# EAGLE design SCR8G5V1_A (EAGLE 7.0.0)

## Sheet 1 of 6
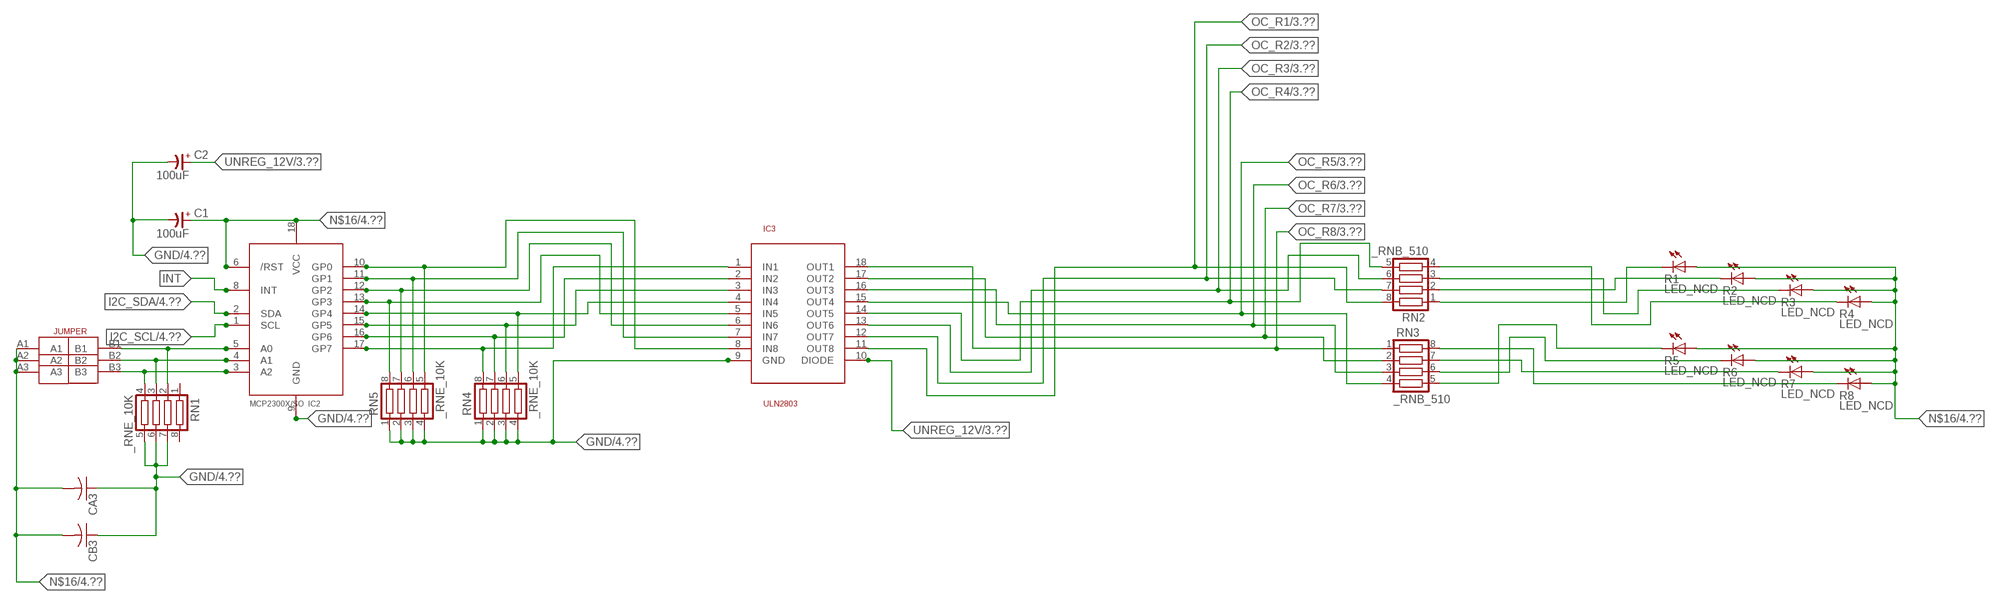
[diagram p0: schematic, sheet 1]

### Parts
C1  100uF  CP-E-025X060  [E-025X060]
C2  100uF  CP-E-025X060  [E-025X060]
CA3  CC1206KRX7R9BB104C1206K  [CC1206KRX7R9BB104]
CB3  TMK316F106ZL-TC1206K  [TMK316F106ZL-T]
IC2  MCP2300X/SO  [SO18W]
IC3  ULN2803  [SO18L]
R1  LED_NCD  [CHIPLED_0603]
R2  LED_NCD  [CHIPLED_0603]
R3  LED_NCD  [CHIPLED_0603]
R4  LED_NCD  [CHIPLED_0603]
R5  LED_NCD  [CHIPLED_0603]
R6  LED_NCD  [CHIPLED_0603]
R7  LED_NCD  [CHIPLED_0603]
R8  LED_NCD  [CHIPLED_0603]
RN1  _RNE_10K  [RNE]
RN2  _RNB_510  [RNB]
RN3  _RNB_510  [RNB]
RN4  _RNE_10K  [RNE]
RN5  _RNE_10K  [RNE]
U$18  JUMPER_3X2  [JUMPER_3X2]

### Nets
GND: C1.- C2.- CA3.1 CB3.1 IC2.9(GND) IC3.9(GND) RN1.5 RN1.6 RN1.7 RN4.1 RN4.2 RN4.3 RN4.4 RN5.1 RN5.2 RN5.3 RN5.4 ; also sheet 4,6
GP4: IC2.14(GP4) IC3.4(IN4) RN4.5
GP6: IC2.16(GP6) IC3.2(IN2) RN4.7
I2C_SCL: IC2.1(SCL) ; also sheet 4
I2C_SDA: IC2.2(SDA) ; also sheet 4
INT: IC2.8(INT)
N$6: IC2.5(A0) RN1.2 U$18.B1
N$7: IC2.4(A1) RN1.3 U$18.B2
N$8: IC2.3(A2) RN1.4 U$18.B3
N$16: C1.+ CA3.2 CB3.2 IC2.6(/RST) IC2.18(VCC) R1.A R2.A R3.A R4.A R5.A R6.A R7.A R8.A U$18.A1 U$18.A2 U$18.A3 ; also sheet 4,6
N$20: R1.C RN2.1
N$21: IC2.12(GP2) IC3.6(IN6) RN5.7
N$22: IC2.11(GP1) IC3.7(IN7) RN5.6
N$23: IC2.10(GP0) IC3.8(IN8) RN5.5
N$29: R2.C RN2.2
N$30: R3.C RN2.3
N$31: R4.C RN2.4
N$32: R8.C RN3.8
N$81: R7.C RN3.7
N$82: R6.C RN3.6
N$83: R5.C RN3.5
N$89: IC2.13(GP3) IC3.5(IN5) RN5.8
N$93: IC2.15(GP5) IC3.3(IN3) RN4.6
N$94: IC2.17(GP7) IC3.1(IN1) RN4.8
OC_R1: IC3.11(OUT8) RN2.8 ; also sheet 3
OC_R2: IC3.12(OUT7) RN2.7 ; also sheet 3
OC_R3: IC3.13(OUT6) RN2.6 ; also sheet 3
OC_R4: IC3.14(OUT5) RN2.5 ; also sheet 3
OC_R5: IC3.15(OUT4) RN3.4 ; also sheet 3
OC_R6: IC3.16(OUT3) RN3.3 ; also sheet 3
OC_R7: IC3.17(OUT2) RN3.2 ; also sheet 3
OC_R8: IC3.18(OUT1) RN3.1 ; also sheet 3
UNREG_12V: C2.+ IC3.10(DIODE) ; also sheet 3,4
Unconnected: RN1.1 RN1.8

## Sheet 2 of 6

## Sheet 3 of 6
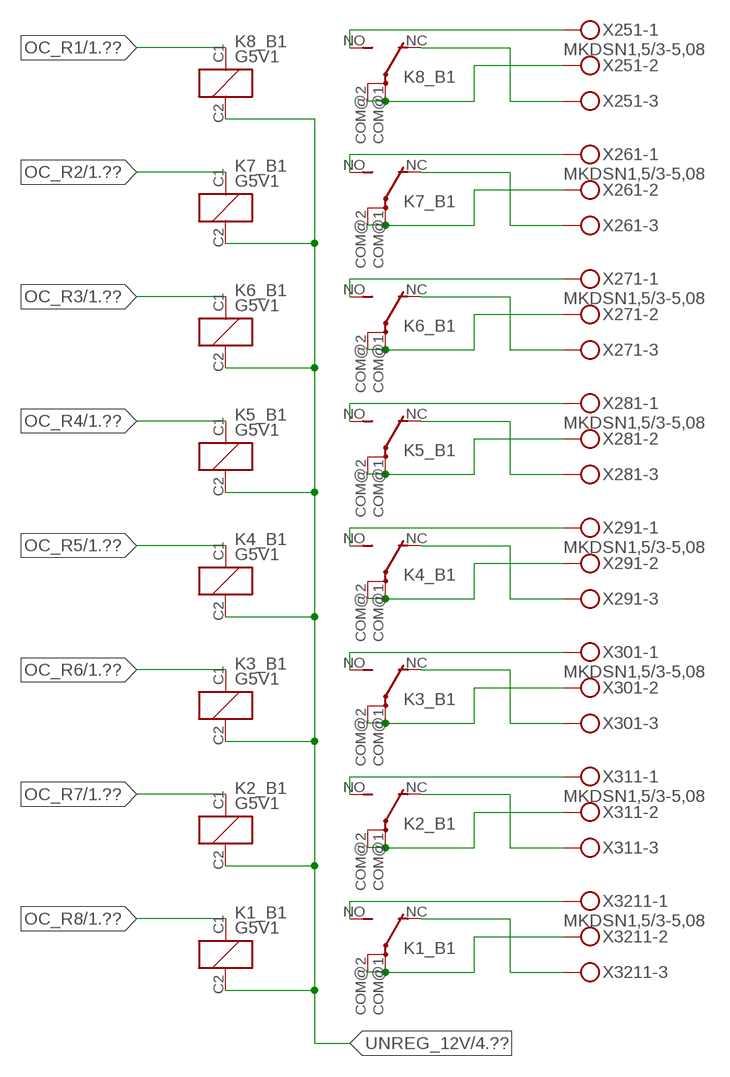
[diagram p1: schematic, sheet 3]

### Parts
K1_B1  G5V1  [G5V1]
K2_B1  G5V1  [G5V1]
K3_B1  G5V1  [G5V1]
K4_B1  G5V1  [G5V1]
K5_B1  G5V1  [G5V1]
K6_B1  G5V1  [G5V1]
K7_B1  G5V1  [G5V1]
K8_B1  G5V1  [G5V1]
X251  MKDSN1,5/3-5,08  [MKDSN1,5/3-5,08]
X261  MKDSN1,5/3-5,08  [MKDSN1,5/3-5,08]
X271  MKDSN1,5/3-5,08  [MKDSN1,5/3-5,08]
X281  MKDSN1,5/3-5,08  [MKDSN1,5/3-5,08]
X291  MKDSN1,5/3-5,08  [MKDSN1,5/3-5,08]
X301  MKDSN1,5/3-5,08  [MKDSN1,5/3-5,08]
X311  MKDSN1,5/3-5,08  [MKDSN1,5/3-5,08]
X3211  MKDSN1,5/3-5,08  [MKDSN1,5/3-5,08]

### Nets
N$203: K8_B1.COM@1(2:P) K8_B1.COM@2(2:P) X251.2
N$204: K8_B1.NC(2:O) X251.3
N$205: K8_B1.NO(2:S) X251.1
N$206: K7_B1.NO(2:S) X261.1
N$207: K6_B1.NO(2:S) X271.1
N$208: K7_B1.NC(2:O) X261.3
N$209: K7_B1.COM@1(2:P) K7_B1.COM@2(2:P) X261.2
N$210: K6_B1.NC(2:O) X271.3
N$211: K6_B1.COM@1(2:P) K6_B1.COM@2(2:P) X271.2
N$212: K5_B1.NC(2:O) X281.3
N$213: K5_B1.COM@1(2:P) K5_B1.COM@2(2:P) X281.2
N$214: K5_B1.NO(2:S) X281.1
N$215: K4_B1.NO(2:S) X291.1
N$216: K4_B1.NC(2:O) X291.3
N$217: K4_B1.COM@1(2:P) K4_B1.COM@2(2:P) X291.2
N$218: K3_B1.NO(2:S) X301.1
N$219: K3_B1.NC(2:O) X301.3
N$220: K3_B1.COM@1(2:P) K3_B1.COM@2(2:P) X301.2
N$221: K2_B1.NO(2:S) X311.1
N$222: K2_B1.NC(2:O) X311.3
N$223: K2_B1.COM@1(2:P) K2_B1.COM@2(2:P) X311.2
N$224: K1_B1.NO(2:S) X3211.1
N$225: K1_B1.NC(2:O) X3211.3
N$226: K1_B1.COM@1(2:P) K1_B1.COM@2(2:P) X3211.2
OC_R1: K8_B1.C1(1:C1) ; also sheet 1
OC_R2: K7_B1.C1(1:C1) ; also sheet 1
OC_R3: K6_B1.C1(1:C1) ; also sheet 1
OC_R4: K5_B1.C1(1:C1) ; also sheet 1
OC_R5: K4_B1.C1(1:C1) ; also sheet 1
OC_R6: K3_B1.C1(1:C1) ; also sheet 1
OC_R7: K2_B1.C1(1:C1) ; also sheet 1
OC_R8: K1_B1.C1(1:C1) ; also sheet 1
UNREG_12V: K1_B1.C2(1:C2) K2_B1.C2(1:C2) K3_B1.C2(1:C2) K4_B1.C2(1:C2) K5_B1.C2(1:C2) K6_B1.C2(1:C2) K7_B1.C2(1:C2) K8_B1.C2(1:C2) ; also sheet 1,4

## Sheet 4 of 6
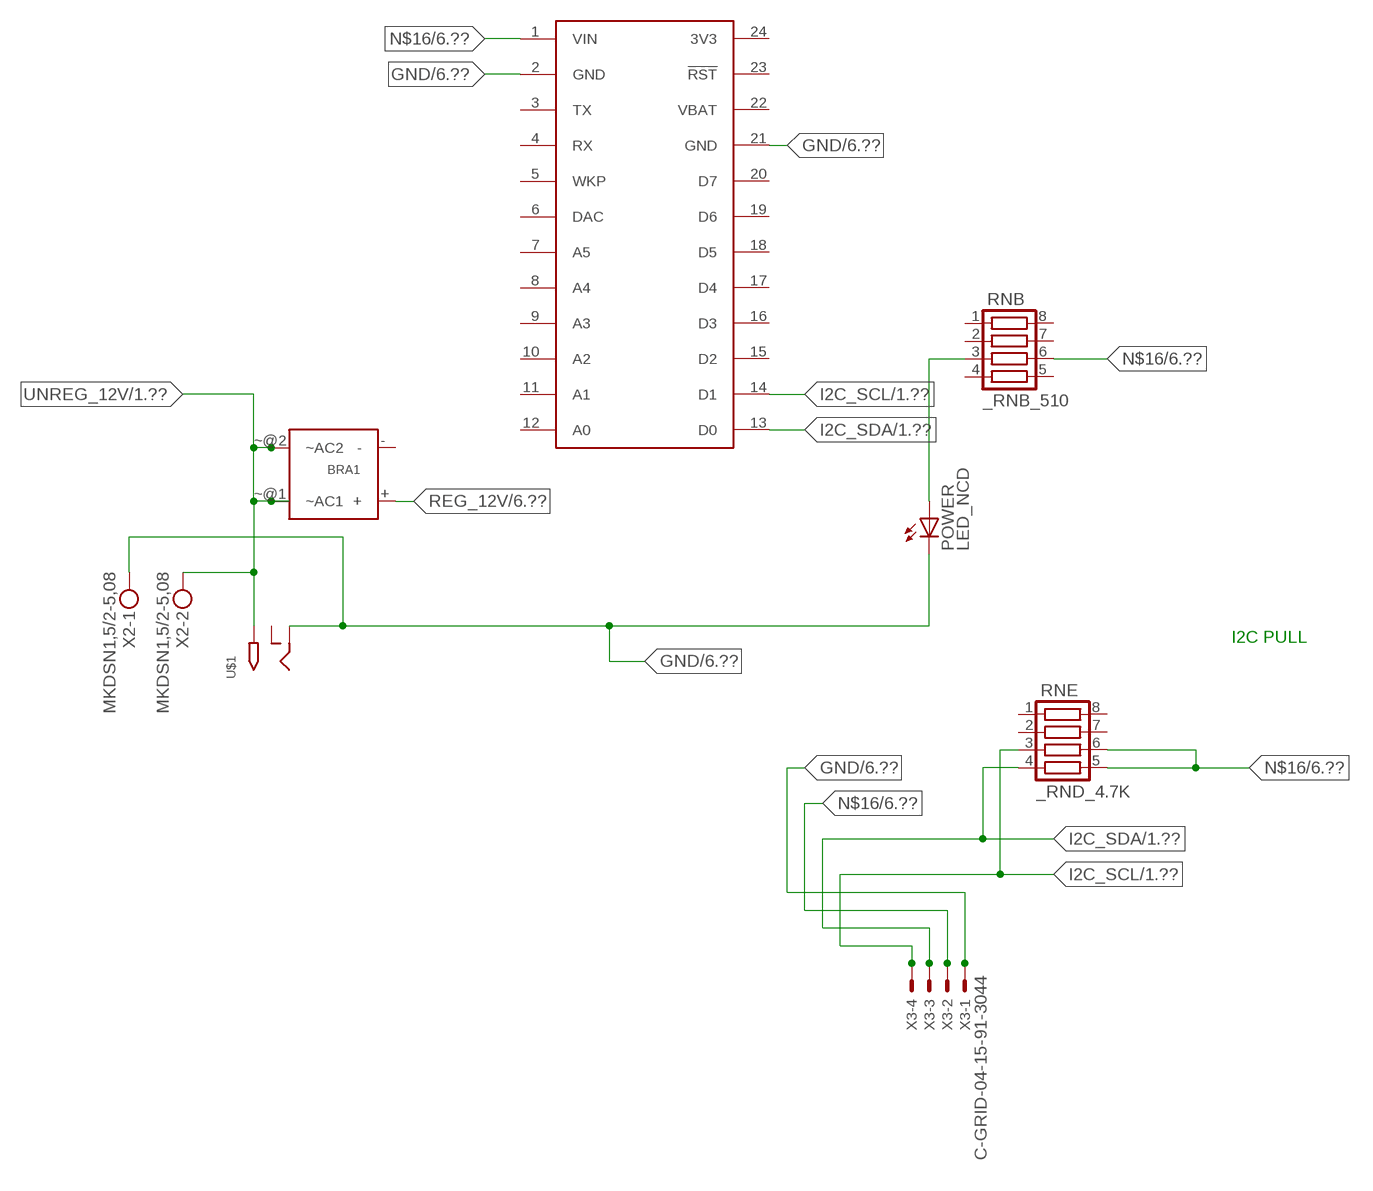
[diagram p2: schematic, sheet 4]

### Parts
BRA1  MB2S_  [MB2S]
POWER  LED_NCD  [CHIPLED_0603]
RNB  _RNB_510  [RNB]
RNE  _RND_4.7K  [RND]
S1  SPARK_CORECORE  [SPARK_CORE]
U$1  2.1MMJACK  [PJ-102A]
X2  MKDSN1,5/2-5,08  [MKDSN1,5/2-5,08]
X3  C-GRID-04-15-91-3044  [15-91-04]

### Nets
GND: POWER.C S1.2(GND) S1.21(GND) U$1.RING X2.1 X3.1 ; also sheet 1,6
I2C_SCL: RNE.3 S1.14(D1) X3.4 ; also sheet 1
I2C_SDA: RNE.4 S1.13(D0) X3.3 ; also sheet 1
N$2: POWER.A RNB.3
N$16: RNB.6 RNE.5 RNE.6 S1.1(VIN) X3.2 ; also sheet 1,6
REG_12V: BRA1.+ ; also sheet 6
UNREG_12V: BRA1.~@1(~AC1) BRA1.~@2(~AC2) U$1.TIP X2.2 ; also sheet 1,3
Unconnected: BRA1.- RNB.1 RNB.2 RNB.4 RNB.5 RNB.7 RNB.8 RNE.1 RNE.2 RNE.7 RNE.8 S1.3(TX) S1.4(RX) S1.5(WKP) S1.6(DAC) S1.7(A5) S1.8(A4) S1.9(A3) S1.10(A2) S1.11(A1) S1.12(A0) S1.15(D2) S1.16(D3) S1.17(D4) S1.18(D5) S1.19(D6) S1.20(D7) S1.23(!RST) U$1.RING_SW

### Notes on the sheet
- I2C PULL

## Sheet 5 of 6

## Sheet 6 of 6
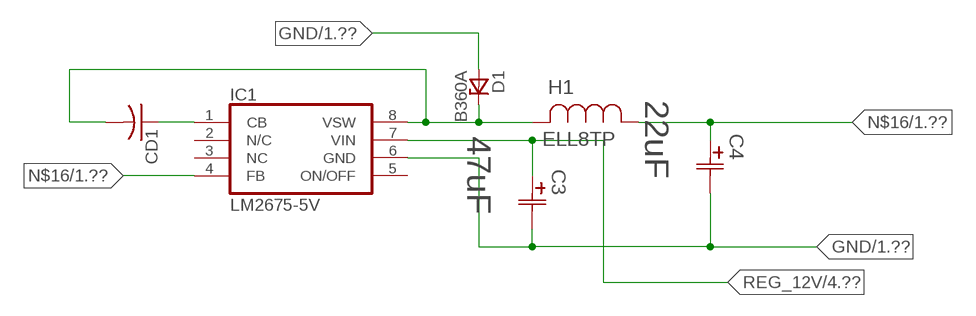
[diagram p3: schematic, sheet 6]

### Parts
C3  47uF  490-5463-6-NDCAP  [C2917(7343)-Y]
C4  22uF  490-5463-6-NDCAP  [C2917(7343)-Y]
CD1  _CD_10NF_50VC1206K  [_CD_10NF_50V]
D1  B360A  [DO214AC_ZENER]
H1  ELL8TP  [IND_ELL8TP]
IC1  LM2675-5V  LM2675  [SO-8]

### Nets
GND: C3.2(C2) C4.2(C2) D1.A IC1.6(GND) ; also sheet 1,4
N$1: CD1.2 D1.C H1.2 IC1.8(VSW)
N$3: CD1.1 IC1.1(CB)
N$16: C4.1(C1) H1.1 IC1.4(FB) ; also sheet 1,4
REG_12V: C3.1(C1) IC1.7(VIN) ; also sheet 4
Unconnected: IC1.2(N/C) IC1.5(ON/OFF)

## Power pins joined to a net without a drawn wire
3V3: S1.24(3V3)
NC: IC1.3(NC)
VBAT: S1.22(VBAT)

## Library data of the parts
BRA1 = NCD_ULTIMATE_LIBRARY:MB2S: Bridge Rectifier BRA MB2S 200V 500ma Digikey MB2S-TPMSTR-ND/MB2S-TP
C1 C2 = NCD_ULTIMATE_LIBRARY:CP-: Capacitors All Kinds POLARIZED CAP
C3 C4 = NCD_ULTIMATE_bhaskar:490-5463-6-ND: NCD CAP
CA3 = NCD_ULTIMATE_LIBRARY:CC1206KRX7R9BB104: Capacitor CA .1uF 50V SMT C1206K CC1206KRX7R9BB104
CB3 = NCD_ULTIMATE_LIBRARY:TMK316F106ZL-T: Capacitor CB 10uF SMT 1206 TMK316F106ZL-T
CD1 = NCD_ULTIMATE_LIBRARY:_CD_10NF_50V: Capacitor 10nF SMT
D1 = NCD_ULTIMATE_bhaskar:B360A: NCD DIODE B350A/B360A
H1 = NCD_ULTIMATE_bhaskar:ELL8TP: NCD coil
IC1 = NCD_ULTIMATE_bhaskar:LM2675: LM2675 NCD http://www.ti.com/lit/ds/symlink/lm2675.pdf
IC2 = NCD_ULTIMATE_LIBRARY:MCP2300X: Semiconductor Port Expander I/O 8-Bit I2C MCP23008 Inexpensive i2c i/o expander - 8 general purpose i/o pins with optional pullups
IC3 = NCD_ULTIMATE_LIBRARY:ULN2803: Semiconductor 8 O.C. N-Channel Transistor Driver Digikey ULN2803AFWGCELTR-ND/ULN2803AFWG,C,EL
K1_B1 K2_B1 K3_B1 K4_B1 K5_B1 K6_B1 K7_B1 K8_B1 = NCD_ULTIMATE_LIBRARY:G5V1: RELAY 1 x switch, 0.5 A/125 V AC, 1 A/24 V DC , Omron
POWER = NCD_ULTIMATE_bhaskar:LED_NCD
R1-R8 = NCD_ULTIMATE_LIBRARY:LED_NCD: LED Digikey 754-1132-2-ND/APT2012SRCPRV
RN1 RN4 RN5 = NCD_ULTIMATE_LIBRARY:_RNE_10K: Resistor Array RNE SMT 10K x 4 Single Resistor Source: http://www.ctscorp.com/components/Datasheets/CTSChipArrayDs.pdf Digikey 742C083103JPTR-ND/742C083103JP; OC_FARNELL: unknown; OC_NEWARK: unknown
RN2 RN3 RNB = NCD_ULTIMATE_LIBRARY:_RNB_510: Resistor Array RNB SMT 510 x 4 Single Resistor Source: http://www.ctscorp.com/components/Datasheets/CTSChipArrayDs.pdf Digikey 742C083511JPTR-ND/ 742C083511JP; OC_FARNELL: unknown; OC_NEWARK: unknown
RNE = NCD_ULTIMATE_LIBRARY:_RND_4.7K: Resistor Array RND SMT 4.7K x 4 Single Resistor Source: http://www.ctscorp.com/components/Datasheets/CTSChipArrayDs.pdf Digikey 742C083472JPTR-ND/742C083472JP; OC_FARNELL: unknown; OC_NEWARK: unknown
S1 = Spark:SPARK_CORE
U$1 = NCD_ULTIMATE_CONNECTORS:2.1MMJACK: 2.1mm x 5.5mm DC jack with internal switch. Digikey part #PJ-102A, 4UCON part #05537 By microbuilder.eu
U$18 = NCD_ULTIMATE_CONNECTORS:JUMPER_3X2
X2 = NCD_ULTIMATE_CONNECTORS:MKDSN1,5/2-5,08: MKDSN 1,5/ 2-5,08 Printklemme
X3 = NCD_ULTIMATE_CONNECTORS:C-GRID-04: CONNECTOR 4-Pos I2C wire to board 2.54 mm (0.100") pitch header Digikey WM1342-ND/0015912045; OC_FARNELL: unknown; OC_NEWARK: unknown
X251 X261 X271 X281 X291 X301 X311 X3211 = NCD_ULTIMATE_CONNECTORS:MKDSN1,5/3-5,08: MKDSN 1,5/ 3-5,08 Printklemme Nennstrom: 13,5 A Nennspannung: 250 V Rastermaß: 5,08 mm Polzahl: 3 Anschlussart: Schraubanschluss Montage: Löten Anschlussrichtung Leiter/Platine: 0 ° Artikelnummer: 1729131 Source: http://eshop.phoenixcontact.com .. 1729131.pdf

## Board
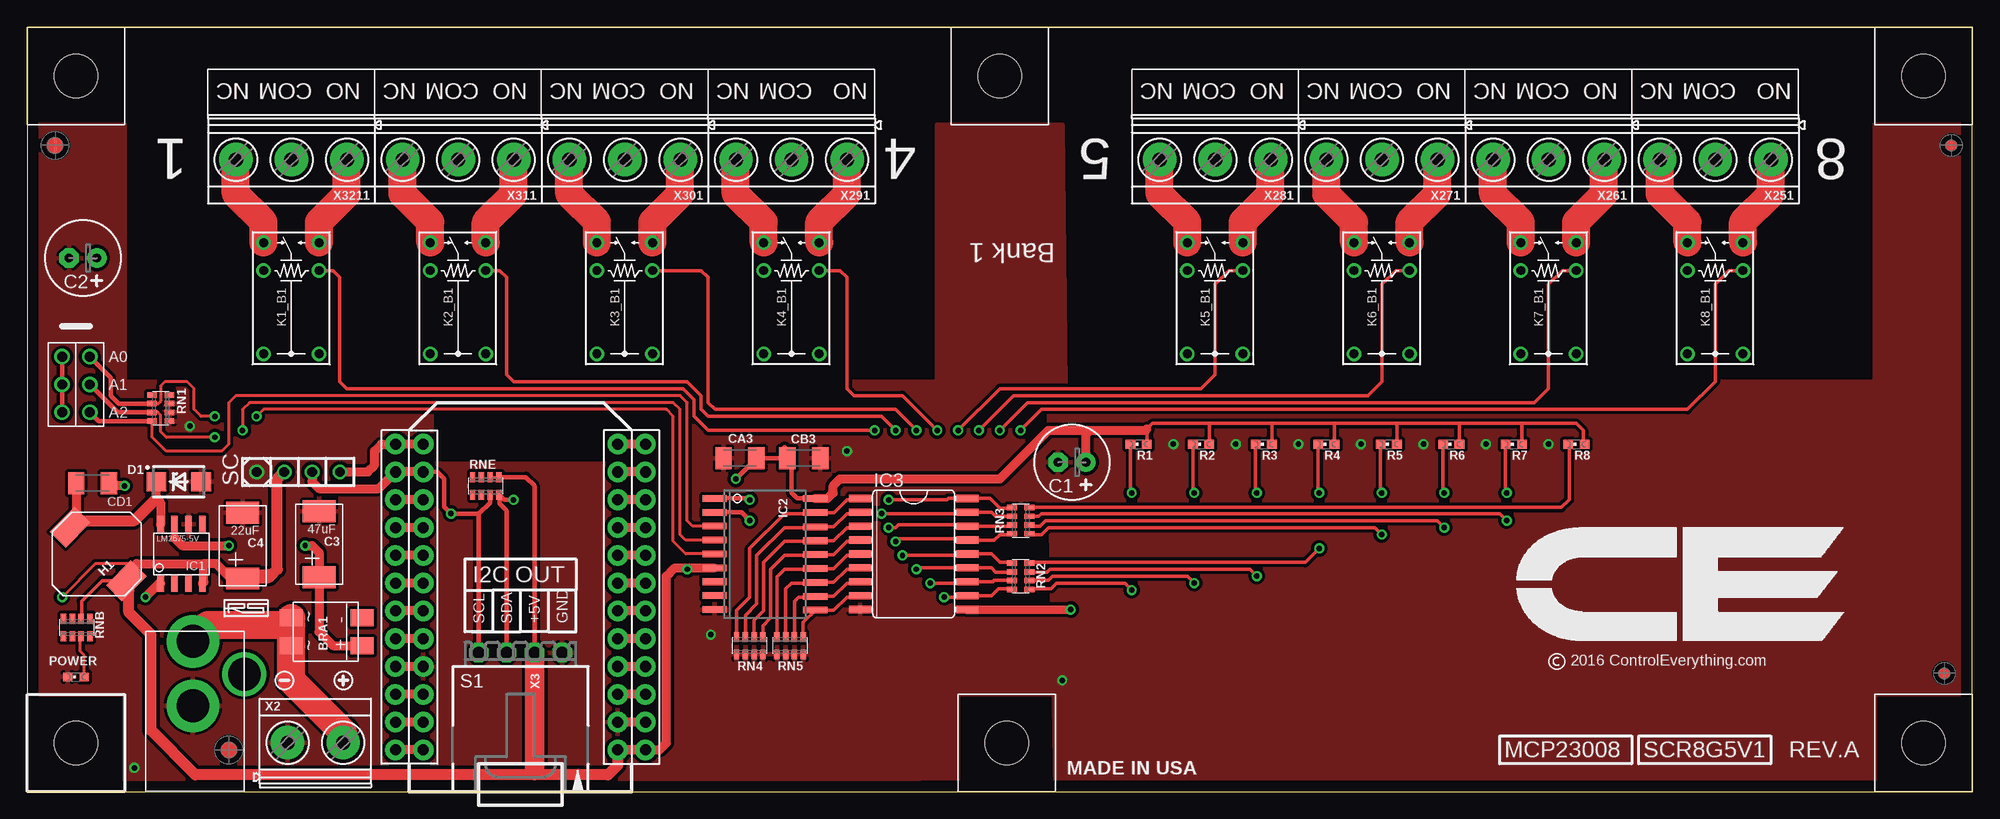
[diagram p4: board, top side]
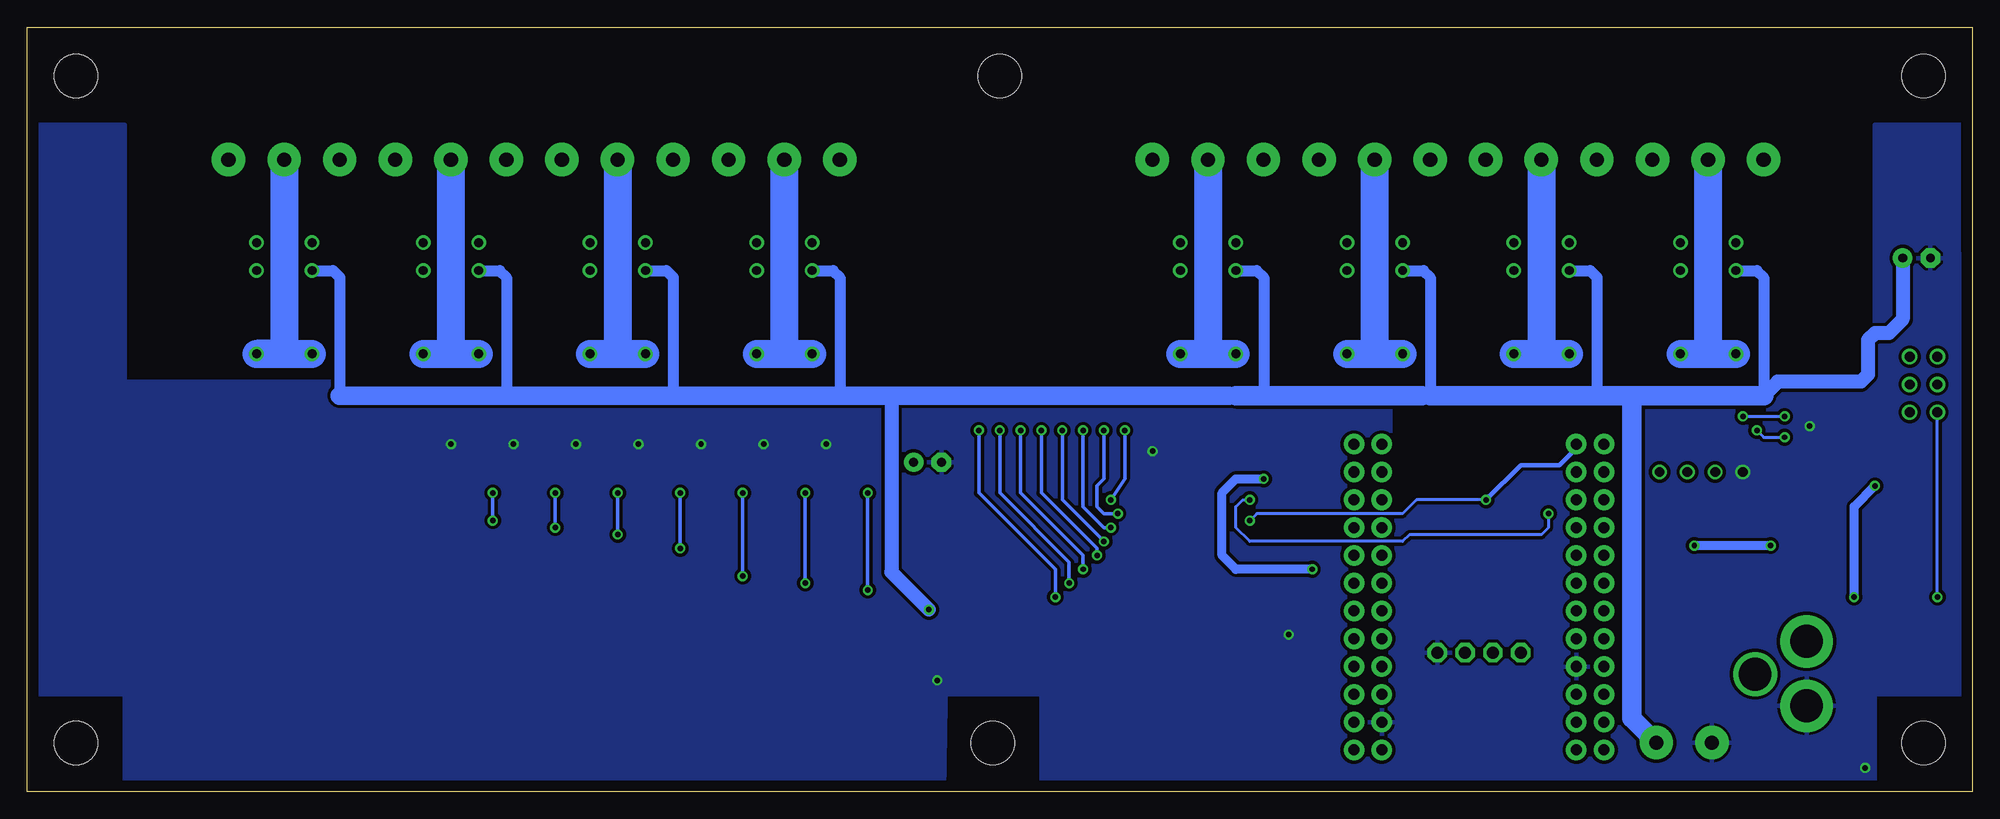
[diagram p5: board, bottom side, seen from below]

Size 177.8 x 69.85 mm. Coordinates in mm from the lower left corner, seen from the top.
Outline: 81.92,0 83.17,0
Outline: 0,50.47 0,49.53
Outline: 0,49.53 0,0 81.92,0
Outline: 81.92,0 177.8,0 177.8,69.85 0,69.85 0,49.53
Copper layers (1*16): Top 0.035mm / dielectric 1.5mm / Bottom 0.035mm
Design rules "default": minimum track width 10mil, minimum drill 24mil, track to track 8mil, track to pad 8mil, pad to pad 8mil, via to via 8mil, smd to smd 8mil, copper to edge 40mil, drill to drill 8mil, minimum pad ring 10mil, minimum via ring 8mil, stop-mask expansion 4mil, vias tented up to drill 0mil, thermal gap 10mil
Holes 3.96 mm at 4.45,4.45

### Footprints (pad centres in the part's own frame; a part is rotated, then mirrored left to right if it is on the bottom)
MB2S = smd 1.55 x 2.1: + 0,-6.5; - 2.54,-6.5; ~@1 0,0; ~@2 2.54,0
E-025X060 = drill 0.813 pad 1.778: + -1.27,0 | drill 0.813 pad 1.778 octagon: - 1.27,0
C2917(7343)-Y = smd 2 x 3: 1 -3,0; 2 3,0
CC1206KRX7R9BB104 = smd 1.5 x 2: 1 -1.5,0; 2 1.5,0
TMK316F106ZL-T = smd 1.5 x 2: 1 -1.5,0; 2 1.5,0
_CD_10NF_50V = smd 1.5 x 2: 1 -1.5,0; 2 1.5,0
DO214AC_ZENER = smd 1.8 x 1.7: A 2.05,0; C -2.05,0
IND_ELL8TP = smd 2.054 x 3.2 rotated 45: 1 -2.442,-2.696; 2 2.442,2.442
SO-8 = smd 0.6 x 1.55: 1 -1.905,-2.69; 2 -0.635,-2.69; 3 0.635,-2.69; 4 1.905,-2.69; 5 1.905,2.71; 6 0.635,2.71; 7 -0.635,2.71; 8 -1.905,2.71
SO18W = smd 0.6 x 2.2: 1 -4.445,-4.6; 2 -3.175,-4.6; 3 -1.905,-4.6; 4 -0.635,-4.6; 5 0.635,-4.6; 6 1.905,-4.6; 7 3.175,-4.6; 8 4.445,-4.6; 9 5.715,-4.6; 10 5.775,4.6; 11 4.505,4.6; 12 3.235,4.6; 13 1.965,4.6; 14 0.695,4.6; 15 -0.575,4.6; 16 -1.845,4.6; 17 -3.145,4.6; 18 -4.445,4.6
SO18L = smd 0.66 x 2.032: 1 -5.08,-4.902; 2 -3.81,-4.902; 3 -2.54,-4.902; 4 -1.27,-4.902; 5 0,-4.902; 6 1.27,-4.902; 7 2.54,-4.902; 8 3.81,-4.902; 9 5.08,-4.902; 10 5.08,4.902; 11 3.81,4.902; 12 2.54,4.902; 13 1.27,4.902; 14 0,4.902; 15 -1.27,4.902; 16 -2.54,4.902; 17 -3.81,4.902; 18 -5.08,4.902
G5V1 = drill 0.813: C1 -2.54,2.54; C2 -2.54,-2.54; COM@1 5.08,-2.54; COM@2 5.08,2.54; NC -5.08,-2.54; NO -5.08,2.54
CHIPLED_0603 = smd 0.8 x 0.8: A 0,-0.75; C 0,0.75
CHIPLED_0603' = smd 0.8 x 0.876: A 0,-0.75; C 0,0.75
RNE = smd 0.5 x 0.9: 1 -1.2,-0.8; 2 -0.4,-0.8; 3 0.4,-0.8; 4 1.2,-0.8; 5 1.2,0.8; 6 0.4,0.8; 7 -0.4,0.8; 8 -1.2,0.8
RNB = smd 0.5 x 0.9: 1 -1.2,-0.8; 2 -0.4,-0.8; 3 0.4,-0.8; 4 1.2,-0.8; 5 1.2,0.8; 6 0.4,0.8; 7 -0.4,0.8; 8 -1.2,0.8
RND = smd 0.5 x 0.9: 1 -1.2,-0.8; 2 -0.4,-0.8; 3 0.4,-0.8; 4 1.2,-0.8; 5 1.2,0.8; 6 0.4,0.8; 7 -0.4,0.8; 8 -1.2,0.8
SPARK_CORE = drill 1.016 pad 1.88: 1 -8.89,13.97; 2 -8.89,11.43; 3 -8.89,8.89; 4 -8.89,6.35; 5 -8.89,3.81; 6 -8.89,1.27; 7 -8.89,-1.27; 8 -8.89,-3.81; 9 -8.89,-6.35; 10 -8.89,-8.89; 11 -8.89,-11.43; 12 -8.89,-13.97; 13 8.89,-13.97; 14 8.89,-11.43; 15 8.89,-8.89; 16 8.89,-6.35; 17 8.89,-3.81; 18 8.89,-1.27; 19 8.89,1.27; 20 8.89,3.81; 21 8.89,6.35; 22 8.89,8.89; 23 8.89,11.43; 24 8.89,13.97; 25 -11.43,13.97; 26 -11.43,11.43; 27 -11.43,8.89; 28 -11.43,6.35; 29 -11.43,3.81; 30 -11.43,1.27; 31 -11.43,-1.27; 32 -11.43,-3.81; 33 -11.43,-6.35; 34 -11.43,-8.89; 35 -11.43,-11.43; 36 -11.43,-13.97; 37 11.43,13.97; 38 11.43,11.43; 39 11.43,8.89; 40 11.43,6.35; 41 11.43,3.81; 42 11.43,1.27; 43 11.43,-1.27; 44 11.43,-3.81; 45 11.43,-6.35; 46 11.43,-8.89; 47 11.43,-11.43; 48 11.43,-13.97
PJ-102A = drill 3 pad 4.8: RING 0.1,-3.39; TIP 0.1,-9.29 | drill 3 pad 3.251: RING_SW -4.6,-6.29
PCB_MOUNTING_HOLE = hole 3.962: 4.445,4.445
JUMPER_3X2 = drill 0.9: A1 0,5.08; A2 0,2.54; A3 0,0; B1 2.54,5.08; B2 2.54,2.54; B3 2.54,0
MKDSN1,5/2-5,08 = drill 1.3 pad 3.048: 1 -2.561,0.025; 2 2.519,0.025
15-91-04 = drill 1.1 pad 1.778 octagon: 1 -3.81,-7.62; 2 -1.27,-7.62; 3 1.27,-7.62; 4 3.81,-7.62
MKDSN1,5/3-5,08 = drill 1.3 pad 3.048: 1 -7.641,0.025; 2 -2.561,0.025; 3 2.519,0.025

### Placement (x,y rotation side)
BRA1  24.13,13.34 90 top
C1  95.5,30.1 180 top
C2  5.08,48.77 180 top
C3  26.67,22.61 90 top
C4  19.68,22.48 90 top
CA3  65.15,30.48 0 top
CB3  70.99,30.48 180 top
CD1  5.97,28.19 180 top
D1  13.84,28.32 0 top
H1  6.35,21.72 90 top
IC1  14.1,21.72 0 top
IC2  67.44,22.35 270 top
IC3  81.03,21.72 270 top
K1_B1  24.13,45.08 270 top
K2_B1  39.37,45.08 270 top
K3_B1  54.61,45.08 270 top
K4_B1  69.85,45.08 270 top
K5_B1  108.58,45.08 270 top
K6_B1  123.83,45.08 270 top
K7_B1  139.06,45.08 270 top
K8_B1  154.31,45.08 270 top
POWER  4.45,10.48 90 top
R1  LED_NCD  [CHIPLED_0603']  101.6,31.75 90 top
R2  LED_NCD  [CHIPLED_0603']  107.31,31.75 90 top
R3  LED_NCD  [CHIPLED_0603']  113.03,31.75 90 top
R4  LED_NCD  [CHIPLED_0603']  118.75,31.75 90 top
R5  LED_NCD  [CHIPLED_0603']  124.46,31.75 90 top
R6  LED_NCD  [CHIPLED_0603']  130.18,31.75 90 top
R7  LED_NCD  [CHIPLED_0603']  135.89,31.75 90 top
R8  LED_NCD  [CHIPLED_0603']  141.6,31.75 90 top
RN1  12.19,35.05 270 top
RN2  90.81,19.69 90 top
RN3  90.81,24.77 270 top
RN4  66.04,13.34 0 top
RN5  69.72,13.34 0 top
RNB  4.51,14.99 0 top
RNE  41.91,27.94 0 top
S1  45.09,17.78 180 top
U$1  15.24,4.45 180 top
U$4  [VISION_REF10]  175.26,10.79 270 top
U$5  PCB_MOUNTING_HOLE  [PCB_MOUNTING_HOLE]  177.8,60.96 90 top
U$6  PCB_MOUNTING_HOLE  [PCB_MOUNTING_HOLE]  93.98,0 90 top
U$7  PCB_MOUNTING_HOLE  [PCB_MOUNTING_HOLE]  93.34,60.96 90 top
U$8  PCB_MOUNTING_HOLE  [PCB_MOUNTING_HOLE]  8.89,60.96 90 top
U$10  [VISION_REF15]  18.41,3.81 0 top
U$11  PCB_MOUNTING_HOLE  [PCB_MOUNTING_HOLE]  177.8,0 90 top
U$12  PCB_MOUNTING_HOLE  [PCB_MOUNTING_HOLE]  177.8,60.96 90 top
U$15  [VISION_REF15]  2.54,59.05 270 top
U$18  3.17,34.67 0 top
U$21  [ICON_USA]  95,1.52 0 top
U$22  [ICON_MINUS]  23.5,10.16 180 top
U$24  [ICON_PLUS]  28.89,10.16 90 top
U$28  [VISION_REF10]  175.9,59.05 270 top
X2  26.35,4.45 0 top
X3  45.09,5.08 180 top
X251  151.76,57.78 180 top
X261  136.53,57.78 180 top
X271  121.28,57.78 180 top
X281  106.05,57.78 180 top
X291  67.31,57.78 180 top
X301  52.07,57.78 180 top
X311  36.83,57.78 180 top
X3211  21.59,57.78 180 top

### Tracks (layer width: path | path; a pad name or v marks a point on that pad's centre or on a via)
GND  (via drill 0.5, 0.9)
  other vias: 14.86,33.4 62.48,14.35 127.64,31.75 94.61,10.16 133.35,31.75 139.06,31.75 121.92,31.75 116.2,31.75 110.49,31.75 104.78,31.75 74.93,31.12 9.78,2.16 20.95,29.21
  pour Bottom (isolate 0.305): -1.91,8.89 8.89,8.89 8.89,0 85.09,0 85.09,8.89 95.25,8.89 94.61,60.96 83.19,60.96 83.19,37.46 8.89,37.46 8.89,60.96 -1.91,60.96
  pour Top (isolate 0.305): -3.81,8.89 8.89,8.89 8.89,0 85.09,0 85.09,8.89 95.25,8.89 94.61,60.96 83.19,60.96 83.19,37.46 8.89,37.46 8.89,60.96 -3.81,60.96
  pour Top (isolate 0.305): 93.34,37.46 168.91,37.46 168.91,60.96 179.71,60.96 179.71,8.89 168.91,8.89 168.91,0 93.98,0
  pour Bottom (isolate 0.305): 93.98,0 93.34,37.46 168.91,37.46 168.91,60.96 182.25,60.96 182.25,8.89 168.91,8.89 168.91,0
GP4
  Top 0.305: RN4.5 67.24,15.17 67.94,15.88 67.94,20.32 69.22,21.59 71.97,21.59 IC2.14 73.73,21.66 74.93,22.86 76,22.86 IC3.4
GP6
  Top 0.305: RN4.7 65.64,16.11 66.67,17.14 66.67,21.59 69.22,24.13 71.97,24.13 IC2.16 73.73,24.2 74.93,25.4 76,25.4 IC3.2
I2C_SCL  (via drill 0.5, 0.9)
  Top 0.406: IC2.1 65.91,26.8 v66.04,26.67 | X3.4 41.27,25.4 | 41.27,25.4 42.29,26.42 42.29,27.12 RNE.3 | S1.14 37.47,29.21 38.1,28.57 38.1,26.04 v38.73,25.4 41.27,25.4
  Top 0.813: v26.04,29.21 26.04,28.32 26.67,27.69 32.13,27.69 33.66,29.21
  Bottom 0.254: v38.73,25.4 38.73,24.13 39.37,23.5 51.44,23.5 52.07,22.86 66.04,22.86 67.31,24.13 67.31,26.04 66.67,26.67 v66.04,26.67
I2C_SDA  (via drill 0.5, 0.9)
  Top 0.406: IC2.2 65.28,25.53 v66.04,24.77 | X3.3 43.81,25.65 43.18,26.29 43.18,27.07 RNE.4 43.58,26.67 v44.45,26.67
  Top 0.813: v28.57,29.21 31.11,29.21 31.75,29.85 31.75,31.12 32.38,31.75 33.66,31.75
  Bottom 0.254: v44.45,26.67 50.8,26.67 52.07,25.4 65.41,25.4 v66.04,24.77
  Bottom 0.406: S1.13 36.2,31.37 37.72,29.85 41.27,29.85 v44.45,26.67
N$1
  Top 0.813: H1.2 3.88,24.77 | D1.C 11.79,26.78 12.19,26.38 IC1.8 | CD1.2 4.47,24.79 4.45,24.77
  Top 1.016: 3.88,24.77 4.45,24.77 9.78,24.77 11.79,26.78
N$2
  Top 0.254: POWER.A 5.2,12.46 4.83,12.83 4.83,14.1 RNB.3
  Top 0.406: 4.95,14.14 RNB.3
N$3  (via drill 0.5)
  Top 0.813: IC1.1 12.04,19.03 v10.79,17.78 | v8.89,27.94 7.72,27.94 CD1.1
  Bottom 0.813: v10.79,17.78 10.79,26.04 v8.89,27.94
N$6  (via drill 0.5)
  Top 0.254: IC2.5 60.2,21.72 59.05,22.86 59.05,34.29 58.42,34.92 21.59,34.92 v20.95,34.29 | v17.14,34.29 15.88,34.29 15.24,34.92 15.24,36.83 14.61,37.46 12.57,37.46 12.19,37.08 12.19,35.69 11.94,35.43 11.41,35.43 RN1.2
  Top 0.406: RN1.2 8.36,35.45 7.62,36.2 7.62,37.85 U$18.B1
  Bottom 0.254: v20.95,34.29 v17.14,34.29
N$7  (via drill 0.5)
  Top 0.254: IC2.4 60.2,22.99 59.69,23.5 59.69,34.92 59.05,35.56 20.32,35.56 19.68,34.92 v19.68,33.02 | v17.14,32.38 12.7,32.38 12.19,32.89 12.19,34.42 11.94,34.67 11.41,34.67 RN1.3
  Top 0.406: RN1.3 8.27,34.65 U$18.B2
  Bottom 0.254: v19.68,33.02 19.05,32.38 v17.14,32.38
N$8
  Top 0.254: IC2.3 60.83,24.26 60.33,24.77 60.33,35.56 59.69,36.2 19.05,36.2 18.41,35.56 18.41,31.75 17.78,31.12 12.7,31.12 11.43,32.38 11.43,33.81 RN1.4
  Top 0.406: RN1.4 6.53,33.85 U$18.B3
N$16  (via drill 0.5, 0.9)
  Top 0.254: RNE.6 RNE.5 | 9.96,20.83 6.22,20.83 v3.17,17.78 | IC2.6 62.74,20.45 | v60.33,20.32 59.82,20.32 59.69,20.45
  Top 0.305: R1.A 102.35,33.13 102.87,33.66 107.95,33.66 | 107.95,33.66 113.67,33.66 | 113.67,33.66 119.38,33.66 | 119.38,33.66 125.09,33.66 | 125.09,33.66 130.81,33.66 | 130.81,33.66 136.53,33.66 | 136.53,33.66 141.6,33.66 142.24,33.02 142.24,31.87 R8.A | R7.A 136.64,33.54 136.53,33.66 | R6.A 130.93,33.54 130.81,33.66 | R5.A 125.21,33.54 125.09,33.66 | R4.A 119.5,33.54 119.38,33.66 | R3.A 113.78,33.54 113.67,33.66 | R2.A 108.06,33.54 107.95,33.66 | H1.1 6.83,19.28 4.95,17.4 4.95,15.83 RNB.6
  Top 0.406: U$18.A3 U$18.A2 U$18.A1 | IC2.18 70.36,26.8 69.85,27.3 69.85,30.76 CB3.2 CA3.2 65.38,29.19 v64.77,28.57 | 62.71,20.32 IC2.6 | RNE.5 45.55,28.74 46.35,27.94 X3.2
  Top 0.61: 69.22,31.39 CB3.2
  Top 0.813: IC2.18 73.15,26.8 73.66,27.3 73.66,27.94 74.3,28.57 88.9,28.57 93.34,33.02 97.16,33.02 | 97.16,33.02 102.23,33.02 102.35,33.13 | C1.+ 96.77,32.64 97.16,33.02 | 16.13,20.83 9.96,20.83 H1.1 | 16.13,20.83 17.27,20.83 18.41,19.69 20.75,19.69 C4.1 | IC1.4 16.13,19.15 16.13,20.83 | S1.1 57.78,3.81 58.42,4.45 58.42,19.69 59.18,20.45 59.69,20.45 62.74,20.45
  Top 1.016: 46.35,2.16 46.35,1.52 | 46.35,1.52 15.37,1.52 11.3,5.59 11.3,14.35 9.27,16.38 9.27,18.41 H1.1 | 22.05,19.69 22.23,19.69 22.86,20.32 22.86,28.57 v23.5,29.21 | S1.1 53.98,2.41 53.09,1.52 46.35,1.52
  Top 1.27: 20.75,19.69 22.05,19.69
  Top 1.778: X3.2 46.35,2.16
  Bottom 0.254: v3.17,17.78 U$18.A3
  Bottom 0.813: v60.33,20.32 67.31,20.32 68.58,21.59 68.58,27.3 67.31,28.57 v64.77,28.57
N$20  (via drill 0.5)
  Top 0.305: R1.C 100.85,27.42 v100.97,27.3 | v100.97,18.41 100.33,19.05 94.11,19.05 93.6,18.54 91.66,18.54 RN2.1
  Bottom 0.305: v100.97,27.3 v100.97,18.41
N$21
  Top 0.305: RN5.7 69.32,18.52 69.85,19.05 71.97,19.05 IC2.12 73.73,19.12 74.93,20.32 76,20.32 IC3.6
N$22
  Top 0.305: RN5.6 70.12,17.42 70.48,17.78 71.97,17.78 IC2.11 73.73,17.85 74.93,19.05 76,19.05 IC3.7
N$23
  Top 0.254: 71.97,16.51 IC2.10
  Top 0.305: RN5.5 70.92,15.46 IC2.10 73.73,16.58 74.93,17.78 76,17.78 IC3.8
N$29  (via drill 0.5)
  Top 0.305: R2.C 106.56,27.42 v106.68,27.3 | v106.68,19.05 106.05,19.69 93.73,19.69 93.34,19.3 91.62,19.3 RN2.2
  Bottom 0.305: v106.68,27.3 v106.68,19.05
N$30  (via drill 0.5)
  Top 0.305: R3.C 112.28,27.42 v112.39,27.3 | v112.39,19.69 111.76,20.32 93.47,20.32 93.22,20.07 91.62,20.07 RN2.3
  Bottom 0.305: v112.39,27.3 v112.39,19.69
N$31  (via drill 0.5)
  Top 0.305: R4.C 118,27.42 v118.11,27.3 | v118.11,22.23 116.84,20.96 91.67,20.96 RN2.4
  Bottom 0.305: v118.11,27.3 v118.11,22.23
N$32
  Top 0.305: RN3.8 140.26,25.96 140.97,26.67 140.97,31.64 R8.C
N$81  (via drill 0.5)
  Top 0.305: R7.C 135.14,27.42 v135.25,27.3 | v135.25,24.77 134.62,25.4 92.71,25.4 92.46,25.15 91.62,25.15 RN3.7
  Bottom 0.305: v135.25,27.3 v135.25,24.77
N$82  (via drill 0.5)
  Top 0.305: R6.C 129.43,27.42 v129.54,27.3 | v129.54,24.13 128.91,24.77 93.09,24.77 92.58,24.26 91.71,24.26 RN3.6
  Bottom 0.305: v129.54,27.3 v129.54,24.13
N$83  (via drill 0.5)
  Top 0.305: R5.C 123.71,27.42 v123.83,27.3 | v123.83,23.5 123.19,24.13 93.34,24.13 92.71,23.5 91.67,23.5 RN3.5
  Bottom 0.305: v123.83,27.3 v123.83,23.5
N$89
  Top 0.305: RN5.8 68.52,19.63 69.22,20.32 71.97,20.32 IC2.13 73.73,20.39 74.93,21.59 76,21.59 IC3.5
N$93
  Top 0.305: RN4.6 66.44,15.64 67.31,16.51 67.31,20.96 69.22,22.86 71.97,22.86 IC2.15 73.73,22.93 74.93,24.13 76,24.13 IC3.3
N$94
  Top 0.305: RN4.8 64.84,16.58 66.04,17.78 66.04,22.23 69.22,25.4 71.94,25.4 IC2.17 73.76,25.5 74.93,26.67 76,26.67 IC3.1
N$203
  Bottom 2.54: X251.2 154.33,40.03 154.31,40 K8_B1.COM@2 K8_B1.COM@1
N$204
  Top 2.54: K8_B1.NC 151.76,52.07 149.22,54.61 149.22,57.74 X251.3
N$205
  Top 2.54: K8_B1.NO 156.84,52.07 159.38,54.61 159.38,57.74 X251.1
N$206
  Top 2.54: K7_B1.NO 141.6,52.07 144.15,54.61 144.15,57.74 X261.1
N$207
  Top 2.54: K6_B1.NO 126.36,52.07 128.91,54.61 128.91,57.74 X271.1
N$208
  Top 2.54: K7_B1.NC 136.53,52.07 133.99,54.61 133.99,57.74 X261.3
N$209
  Bottom 2.54: K7_B1.COM@2 139.06,40 | 139.06,40 K7_B1.COM@1 | X261.2 139.09,40.03 139.06,40
N$210
  Top 2.54: K6_B1.NC 121.28,52.07 118.75,54.61 118.75,57.74 X271.3
N$211
  Bottom 2.54: K6_B1.COM@2 123.83,40 | 123.83,40 K6_B1.COM@1 | X271.2 123.85,40.03 123.83,40
N$212
  Top 2.54: K5_B1.NC 106.05,52.07 103.5,54.61 103.5,57.74 X281.3
N$213
  Bottom 2.54: K5_B1.COM@2 108.58,40 | 108.58,40 K5_B1.COM@1 | X281.2 108.61,40.03 108.58,40
N$214
  Top 2.54: K5_B1.NO 111.12,52.07 113.67,54.61 113.67,57.74 X281.1
N$215
  Top 2.54: K4_B1.NO 72.39,52.07 74.93,54.61 74.93,57.74 X291.1
N$216
  Top 2.54: K4_B1.NC 67.31,52.07 64.77,54.61 64.77,57.74 X291.3
N$217
  Bottom 2.54: K4_B1.COM@2 69.85,40 | 69.85,40 K4_B1.COM@1 | X291.2 69.87,40.03 69.85,40
N$218
  Top 2.54: K3_B1.NO 57.15,52.07 59.69,54.61 59.69,57.74 X301.1
N$219
  Top 2.54: K3_B1.NC 52.07,52.07 49.53,54.61 49.53,57.74 X301.3
N$220
  Bottom 2.54: K3_B1.COM@2 54.61,40 | 54.61,40 K3_B1.COM@1 | X301.2 54.63,40.03 54.61,40
N$221
  Top 2.54: K2_B1.NO 41.91,52.07 44.45,54.61 44.45,57.74 X311.1
N$222
  Top 2.54: K2_B1.NC 36.83,52.07 34.29,54.61 34.29,57.74 X311.3
N$223
  Bottom 2.54: K2_B1.COM@2 39.37,40 | 39.37,40 K2_B1.COM@1 | X311.2 39.39,40.03 39.37,40
N$224
  Top 2.54: K1_B1.NO 26.67,52.07 29.21,54.61 29.21,57.74 X3211.1
N$225
  Top 2.54: K1_B1.NC 21.59,52.07 19.05,54.61 19.05,57.74 X3211.3
N$226
  Bottom 2.54: K1_B1.COM@2 24.13,40 | 24.13,40 K1_B1.COM@1 | X3211.2 24.15,40.03 24.13,40
OC_R1  (via drill 0.5)
  Top 0.305: RN2.8 89.95,18.54 88.77,18.54 88.14,17.91 IC3.11 85.8,17.78 v83.82,17.78 | v90.81,33.02 92.71,34.92 151.76,34.92 154.31,37.46 154.31,46.35 155.57,47.62 K8_B1.C1
  Bottom 0.305: v90.81,33.02 90.81,27.3 83.82,20.32 v83.82,17.78
OC_R2  (via drill 0.5)
  Top 0.305: RN2.7 89.99,19.3 88.39,19.3 88.27,19.18 IC3.12 85.8,19.05 v82.55,19.05 | v88.9,33.02 91.44,35.56 137.79,35.56 139.06,36.83 139.06,46.35 140.34,47.62 K7_B1.C1
  Bottom 0.305: v88.9,33.02 88.9,27.3 82.55,20.96 v82.55,19.05
OC_R3  (via drill 0.5)
  Top 0.305: RN2.6 89.99,20.07 88.52,20.07 88.14,20.45 IC3.13 81.53,20.45 81.41,20.32 v81.28,20.32 | v87,33.02 90.17,36.2 122.56,36.2 123.83,37.46 123.83,46.35 125.09,47.62 K6_B1.C1
  Bottom 0.305: v87,33.02 87,27.3 81.28,21.59 v81.28,20.32
OC_R4  (via drill 0.5)
  Top 0.305: RN2.5 89.94,20.96 88.9,20.96 88.14,21.72 IC3.14 85.8,21.59 v80.01,21.59 | v85.09,33.02 88.9,36.83 107.31,36.83 108.58,38.1 108.58,46.35 109.86,47.62 K5_B1.C1
  Bottom 0.305: v85.09,33.02 85.09,27.3 80.01,22.23 v80.01,21.59
OC_R5  (via drill 0.5)
  Top 0.305: RN3.4 89.94,23.5 88.9,23.5 88.39,22.99 IC3.15 85.8,23.11 79.63,23.11 v79.38,22.86 | v83.19,33.02 80.01,36.2 75.56,36.2 74.93,36.83 74.93,46.99 74.3,47.62 K4_B1.C1
  Bottom 0.305: v83.19,33.02 83.19,26.67 v79.38,22.86
OC_R6  (via drill 0.5)
  Top 0.305: RN3.3 89.9,24.26 IC3.16 85.8,24.38 79.63,24.38 79.38,24.13 v78.74,24.13 | v81.28,33.02 79.38,34.92 62.87,34.92 62.23,35.56 62.23,46.99 61.59,47.62 K3_B1.C1
  Bottom 0.305: v81.28,33.02 81.28,26.04 79.38,24.13 v78.74,24.13
OC_R7  (via drill 0.5)
  Top 0.305: RN3.2 89.99,25.15 88.52,25.15 88.14,25.53 IC3.17 85.8,25.4 v78.11,25.4 | v79.38,33.02 78.11,34.29 62.23,34.29 61.59,34.92 61.59,36.2 60.33,37.46 44.45,37.46 43.81,38.1 43.81,46.99 43.18,47.62 K2_B1.C1
  Bottom 0.305: v79.38,33.02 79.38,28.57 80.01,27.94 80.01,26.04 79.38,25.4 v78.11,25.4
OC_R8  (via drill 0.5)
  Top 0.305: RN3.1 89.95,25.91 88.9,25.91 88.01,26.8 IC3.18 84.2,26.8 84.07,26.67 v78.74,26.67 | v77.47,33.02 62.23,33.02 60.96,34.29 60.96,35.81 59.94,36.83 29.21,36.83 28.57,37.46 28.57,46.99 27.94,47.62 K1_B1.C1
  Bottom 0.305: v77.47,33.02 77.47,28.57 v78.74,26.67
REG_12V  (via drill 0.5)
  Top 0.61: IC1.7 13.46,23.16 | 14.1,22.48 14.15,22.48
  Top 0.813: v18.41,22.48 14.15,22.48 13.46,23.16 | v25.4,22.48 26.04,22.48 26.67,21.84 C3.1 26.67,14.61 27.94,13.34 BRA1.+
  Bottom 0.813: v18.41,22.48 v25.4,22.48
UNREG_12V  (via drill 0.5)
  Top 0.762: v95.38,16.64 IC3.10
  Top 2.54: X2.2 28.87,5.42 24.13,10.16 BRA1.~@1 24.13,15.24 | 24.13,15.24 BRA1.~@2 | U$1.TIP 15.14,13.87 16.51,15.24 24.13,15.24
  Bottom 1.016: K1_B1.C2 19.68,47.62 19.05,46.99 19.05,36.2 | K2_B1.C2 34.92,47.62 34.29,46.99 34.29,36.2 | K3_B1.C2 50.16,47.62 49.53,46.99 49.53,36.2 50.29,36.2 | K4_B1.C2 65.41,47.62 64.77,46.99 64.77,36.2 | 67.31,36.2 67.94,36.2 | K5_B1.C2 104.14,47.62 103.5,46.99 103.5,36.83 104.14,36.2 | 98.81,36.2 99.06,36.2 | K6_B1.C2 119.38,47.62 118.75,46.99 118.75,36.83 118.11,36.2 | 116.84,36.2 116.59,36.2 | K7_B1.C2 134.62,47.62 133.99,46.99 133.99,36.2 | 134.37,36.2 134.62,36.2 | K8_B1.C2 149.86,47.62 149.22,46.99 149.22,36.2
  Bottom 1.27: 98.81,36.2 98.81,20.07 v95.38,16.64 | C2.+ 6.35,43.18 7.62,41.91 8.89,41.91 9.53,41.27 9.53,38.1 10.16,37.46 17.78,37.46 19.05,36.2
  Bottom 1.676: 67.94,36.2 98.81,36.2 | 99.06,36.2 104.14,36.2 116.59,36.2 | 116.84,36.2 118.11,36.2 133.99,36.2 134.37,36.2 | 134.62,36.2 149.22,36.2
  Bottom 1.778: 49.53,36.2 34.29,36.2 31.11,36.2 | 31.11,36.2 19.05,36.2 | 67.31,36.2 64.77,36.2 50.29,36.2 | 31.11,36.2 31.11,6.71 X2.2

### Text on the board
tNames: NC | COM | NO | NC | COM | NO | NC | COM | NO | NC | COM | NO | NC | COM | NO | NC | COM | NO | NC | COM | NO | NC | COM | NO | 1 | 4 | 5 | 8 | Bank 1 | A0 | A1 | A2 | SC | I2C OUT | SCL | SDA | +5V | GND | 2016 ControlEverything.com | MCP23008 | SCR8G5V1 | REV.A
